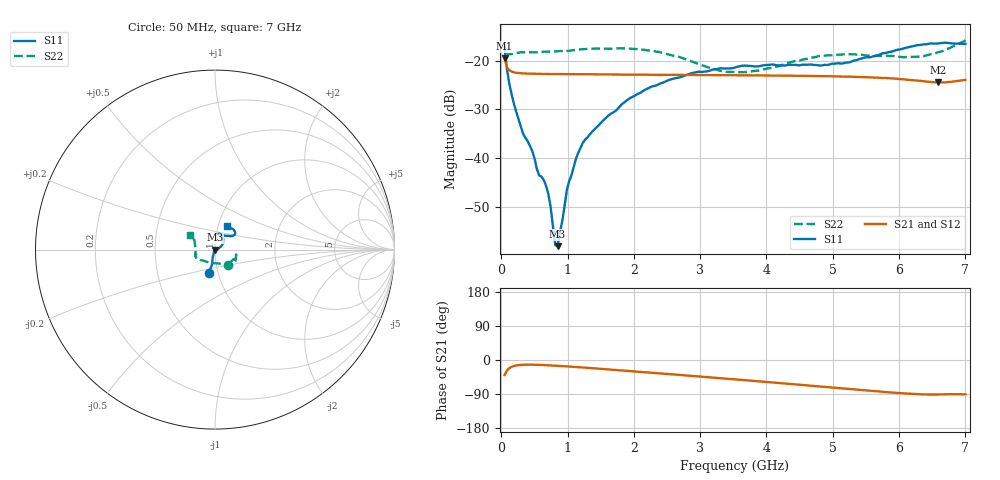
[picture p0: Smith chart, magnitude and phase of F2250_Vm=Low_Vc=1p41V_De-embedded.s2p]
! Integrated Device Technology
! Corporate Headquarters
! 6024 Silver Creek Valley Road
! San Jose, CA 95138  USA
! Phone:  1-408-284-8200
! Toll Free:  1-800-223-1366
! Webpage:  http://www.idt.com/
! Timing and RF Division
! 515 Groton Road, Suite 102
! Westford, MA 01886-6024
! Device:  F2250
! Description: Voltage Variable RF Attenuator
! Frequency:  50.0 -  6000.00 MHz
! Package:  3x3 mm Thin QFN Plastic Package: 16 pin
! Ports:  2 RF, 3 DC
!  Pin  1  = GND
!  Pin  2  = NC
!  Pin  3  = RF1  = Port 1
!  Pin  4  = NC
!  Pin  5  = GND
!  Pin  6  = GND
!  Pin  7  = GND
!  Pin  8  = GND
!  Pin  9  = NC
!  Pin 10  = RF2  = Port 2
!  Pin 11  = NC
!  Pin 12  = GND
!  Pin 13  = GND
!  Pin 14  = VCNTRL
!  Pin 15  = VDD
!  Pin 16  = VMODE
! Vcntrl:  1.410 Volts
! Vmode:  +0.000 Volts
! Vdd:  +3.30  Volts
! Current:  1.193 mA
! Data:  The device was measured on a the F2250 evaluation board which has
!  individual transmission lines to the RF pins.  Data was collected
!  using a calibrated network analyzer.  The evaluation board was
!  de-embedded using a TRL calibration technique.
!  The reference plane is the edge of the package pin.
! Misc:  SN 10
!  Action Tracker AT0258
! Date Measured:  2014-11-26
! Date:  2015-10-15  MJV
! Note:
!  Integrated Device Technology supplies this data as a sample of measured
!  data at the package pin for this product.  Your particular data for this
!  product may vary.
!  Data was taken at 25 degrees C.
!  Integrated Device Technology reserves the right to change this data at anytime.
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# GHz S dB R 50
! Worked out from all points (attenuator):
!   201 points, 50 MHz to 7 GHz, reference 50 ohm
!   highest |S21| = -19.54 dB at 50 MHz (marker M1); lowest = -24.5 dB at 6.583 GHz (marker M2)
!   lowest |S11| = -58.0 dB at 849.2 MHz (marker M3), VSWR 1.00, Z = 50.1 - j0.11 ohm
!   |S11| at or under -10 dB: start of sweep to end of sweep
!   |S22| runs from -22.4 to -15.9 dB; largest |S21 - S12| = 0.00025
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0.05  -17.38 -104.6  -19.54 -39.6  -19.54 -39.6  -19.02 -49.6
0.1195  -24.61 -103.5  -21.96 -21.7  -21.95 -21.7  -18.70 -18.9
0.189  -28.76 -107.1  -22.39 -16.0  -22.40 -16.0  -18.55 -14.4
0.328  -34.95 -110.6  -22.61 -12.6  -22.62 -12.6  -18.28 -13.1
0.467  -38.53 -117.5  -22.68 -12.4  -22.68 -12.4  -18.30 -14.0
0.57125  -43.50 -118.3  -22.70 -12.9  -22.72 -12.9  -18.27 -16.3
0.6755  -45.64 -108.3  -22.74 -13.7  -22.74 -13.7  -18.18 -18.3
0.745  -50.03 -107.6  -22.76 -14.3  -22.75 -14.3  -18.15 -19.9
0.8145  -57.78 -99.9  -22.75 -15.0  -22.75 -15.0  -18.12 -21.5
0.84925  -57.99 -60.9  -22.75 -15.4  -22.76 -15.4  -18.09 -22.4
0.98825  -46.53 -18.6  -22.76 -16.8  -22.79 -16.8  -18.03 -25.0
1.12725  -40.06 4.1  -22.78 -18.4  -22.80 -18.4  -17.82 -27.2
1.2315  -36.78 10.3  -22.79 -19.7  -22.80 -19.7  -17.65 -29.2
1.9265  -27.79 29.7  -22.89 -28.9  -22.86 -28.9  -17.55 -37.5
2.37825  -24.81 38.9  -22.92 -35.0  -22.92 -35.0  -18.22 -43.3
2.93425  -22.37 54.1  -22.94 -42.8  -22.94 -42.8  -20.48 -57.5
3.525  -21.39 68.6  -23.01 -51.1  -23.01 -51.2  -22.33 -94.0
4.7065  -20.88 70.4  -23.13 -68.4  -23.14 -68.4  -19.36 -150.3
5.2625  -20.33 51.7  -23.29 -76.8  -23.32 -76.7  -18.69 -159.2
5.85325  -18.24 38.4  -23.62 -85.3  -23.62 -85.4  -19.06 -169.9
6.583  -16.50 44.4  -24.48 -91.1  -24.47 -91.1  -18.28 159.5
7  -16.56 62.7  -23.93 -90.6  -23.92 -90.7  -15.88 148.6
